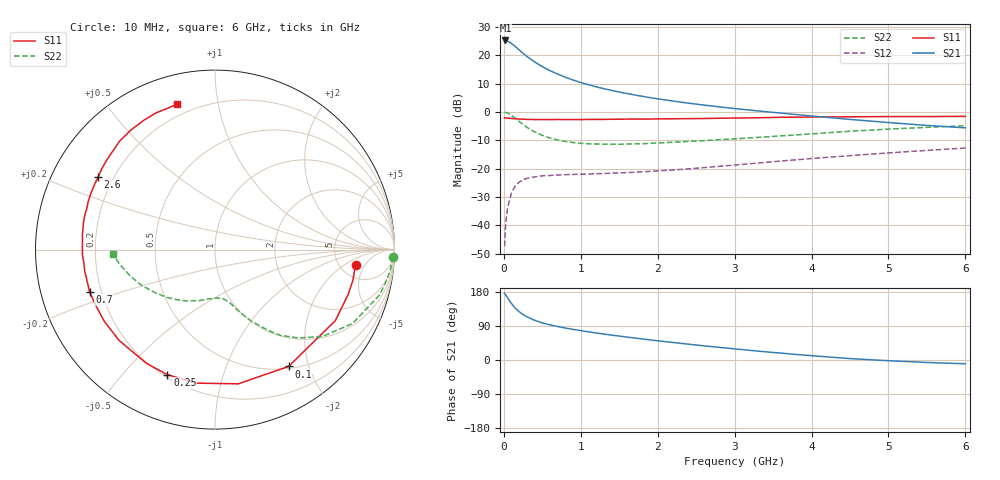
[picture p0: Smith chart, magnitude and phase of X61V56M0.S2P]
! SIEMENS Small Signal Semiconductors
! BFP193W
! Si NPN RF Bipolar Junction Transistor in SOT343
! VCE = 1.5 V  IC = 6 mA
! Common Emitter S-Parameters:  April 1994
# GHz  S  MA  R  50
!  f  S11  S21  S12  S22
! GHz  MAG  ANG  MAG  ANG  MAG  ANG  MAG  ANG
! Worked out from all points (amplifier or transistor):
!   40 points, 10 MHz to 6 GHz, reference 50 ohm
!   highest |S21| = 25.2 dB at 20 MHz (marker M1)
!   |S21| within 3 dB of that: start of sweep to 185.2 MHz
!   unconditionally stable (mu >= 1): 1.537 GHz to 4.696 GHz
!   at 200 MHz: K = 0.16, MSG = 23.3 dB, |S12| = -24.7 dB
!   at 1.5 GHz: K = 0.99, MSG = 14.3 dB, |S12| = -21.5 dB
!   at 6 GHz: K = 0.94, MSG = 3.6 dB, |S12| = -12.7 dB
!   S11 on the Smith chart (normalised r, x): 10 MHz: 7.02, -3.09; 100 MHz: 0.53, -1.69; 250 MHz: 0.21, -0.67; 700 MHz: 0.16, -0.16; 2.6 GHz: 0.14, +0.28; 6 GHz: 0.14, +0.76
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0.01  0.7874 -6.1  18.16 175.9  0.0043 87.4  0.9908 -2.3
0.02  0.7872 -12.5  18.24 173.3  0.0086 83.3  0.9842 -6.4
0.05  0.7785 -30.6  17.7 163.5  0.021 75.5  0.952 -15.3
0.1  0.7692 -57.8  16.12 148.8  0.0376 62.0  0.8697 -28.3
0.15  0.759 -80.1  14.24 136.5  0.0502 51.9  0.7697 -39.0
0.2  0.7508 -97.6  12.39 127.1  0.0581 44.5  0.6773 -46.6
0.25  0.746 -110.8  10.85 119.9  0.0639 38.8  0.6009 -52.7
0.3  0.7399 -121.2  9.524 113.9  0.0673 34.7  0.5352 -56.9
0.4  0.7359 -136.5  7.621 104.8  0.0717 29.5  0.445 -63.2
0.5  0.735 -147.1  6.303 98.0  0.0749 26.4  0.3869 -67.4
0.6  0.7335 -155.0  5.341 92.7  0.0759 24.4  0.3468 -70.7
0.7  0.7373 -161.4  4.661 88.3  0.0773 23.7  0.3197 -73.0
0.9  0.7356 -170.7  3.666 80.7  0.0792 23.2  0.2889 -77.6
1.1  0.7392 -177.7  3.032 74.3  0.0807 23.8  0.2741 -81.8
1.3  0.7397 176.3  2.575 68.5  0.0822 25.2  0.2707 -86.0
1.6  0.748 168.5  2.116 60.4  0.0854 28.0  0.2719 -92.0
2.2  0.759 155.7  1.557 46.2  0.0949 33.9  0.2921 -105.1
2.6  0.7667 148.1  1.324 37.4  0.1044 37.2  0.3115 -113.9
3.2  0.7876 137.7  1.079 25.5  0.1223 40.2  0.349 -126.8
4.5  0.8223 118.9  0.739 3.7  0.1698 39.7  0.4571 -154.4
5.5  0.8297 109.2  0.579 -6.5  0.2098 35.7  0.536 -171.0
6  0.8369 104.8  0.525 -10.0  0.2316 33.4  0.5705 -177.7
